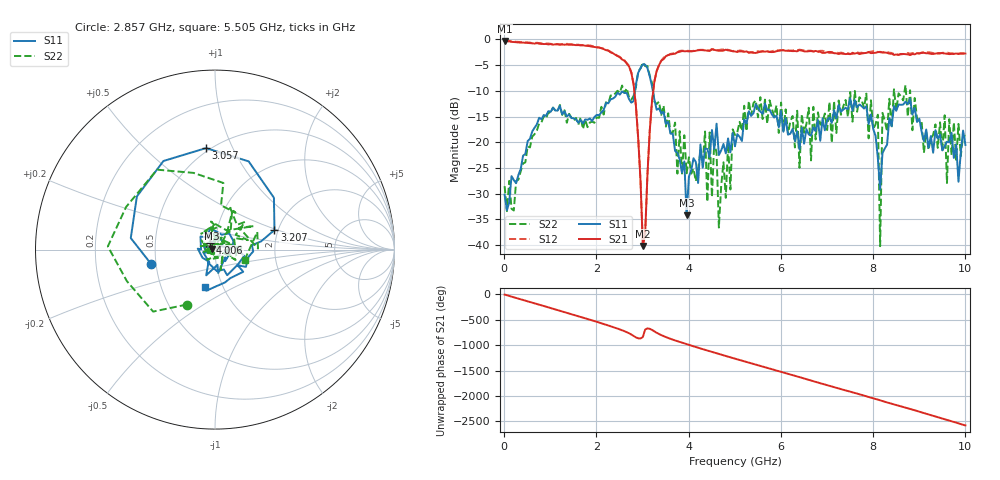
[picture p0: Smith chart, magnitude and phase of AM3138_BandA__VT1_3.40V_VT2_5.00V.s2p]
! Date/Time: Tue, Nov 13, 2018 4:43 PM
! Network Analyzer: Agilent Technologies E8364B Rev: A.07.50.67
! Sweep from 0.010 to 10.000 GHz, 201 Points, Sweep Type: LIN
! Power Supply: 3.401 V, 0.000 A
# Hz S DB R 50
!freq MagS11 AngS11 MagS21 AngS21 MagS12 AngS12 MagS22 AngS22
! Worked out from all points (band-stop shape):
!   201 points, 10 MHz to 10 GHz, reference 50 ohm
!   highest |S21| = -0.31 dB at 10 MHz (marker M1); lowest = -40.2 dB at 3.007 GHz (marker M2)
!   |S21| within 3 dB of the highest: start of sweep to 2.473 GHz; 3.503 GHz to end of sweep
!   lowest |S11| = -34.2 dB at 3.956 GHz (marker M3), VSWR 1.04, Z = 48.2 + j0.52 ohm
!   |S11| at or under -10 dB: start of sweep to 2.838 GHz; 3.224 GHz to end of sweep
!   |S22| runs from -40.2 to -4.5 dB; largest |S21 - S12| = 0.036
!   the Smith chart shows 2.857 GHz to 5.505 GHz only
!   S11 on the Smith chart (normalised r, x): 2.857 GHz: 0.47, -0.09; 3.057 GHz: 0.48, +0.80; 3.207 GHz: 1.91, +0.47; 4.006 GHz: 0.95, +0.07; 5.505 GHz: 0.82, -0.36
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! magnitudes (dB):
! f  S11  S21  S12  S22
! 10 MHz  -30.2  -0.3  -0.2  -28.5
! 1.708 GHz  -16.4  -1.2  -1.1  -17.4
! 2.857 GHz  -8.7  -13.0  -12.9  -9.3
! 3.007 GHz  -4.9  -40.2  -39.9  -4.5
! 3.057 GHz  -4.9  -38.0  -37.9  -5.2
! 3.207 GHz  -9.2  -12.0  -11.8  -8.5
! 3.357 GHz  -13.4  -5.0  -5.0  -12.1
! 3.956 GHz  -34.2  -2.3  -2.2  -26.0
! 4.006 GHz  -26.7  -2.3  -2.2  -22.9
! 4.555 GHz  -21.3  -2.0  -2.0  -19.9
! 4.655 GHz  -22.5  -2.2  -2.1  -36.6
! 5.005 GHz  -20.8  -2.4  -2.2  -18.6
! 5.505 GHz  -13.3  -2.5  -2.3  -15.1
! 6.404 GHz  -21.4  -2.1  -2.0  -25.0
! 6.703 GHz  -17.1  -2.3  -2.4  -13.1
! 8.102 GHz  -23.1  -2.5  -2.4  -14.6
! 8.152 GHz  -29.2  -2.4  -2.5  -40.2
! 8.202 GHz  -22.1  -2.5  -2.6  -14.3
! 8.352 GHz  -15.3  -2.8  -2.6  -11.5
! 9.55 GHz  -20.8  -2.7  -2.6  -14.8
! 9.6 GHz  -19.9  -2.8  -2.6  -27.9
! 10 GHz  -20.5  -2.8  -2.6  -18.8
